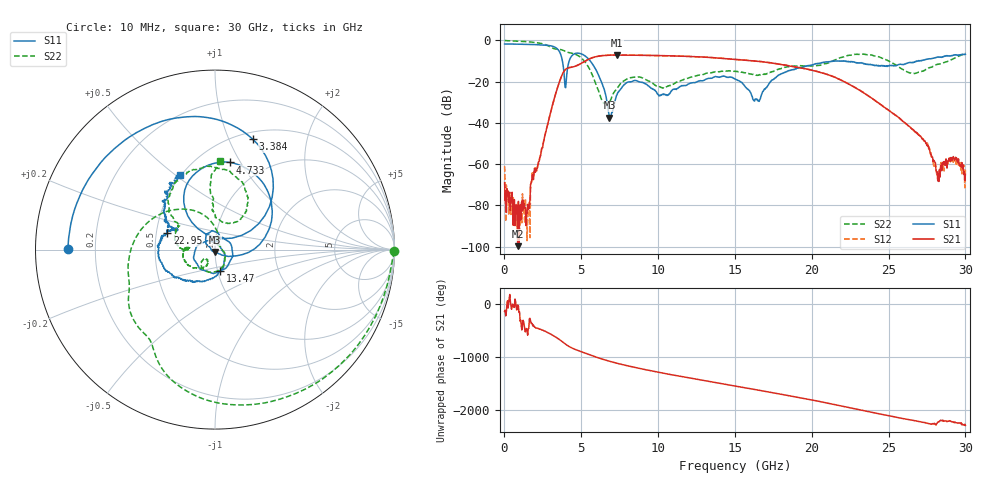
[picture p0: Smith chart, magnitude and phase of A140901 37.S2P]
!  2-Port S-parameters saved by WinCal
! VAR MeasName=S-Parameters (CALIBRATED_DATA) read from VNA (N5244A)
! VAR MeasDate=11/3/2014 9:33:30 AM
! VAR NAME=A140901 37
! VAR FILENAME=A140901 37.S2P
! VAR DATE=11/3/2014 9:33:30 AM
! VAR PHYS_PORTS=1,2
# Hz S RI R 50
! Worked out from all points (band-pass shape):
!   801 points, 10 MHz to 30 GHz, reference 50 ohm
!   highest |S21| = -7.08 dB at 7.32 GHz (marker M1); lowest = -99.8 dB at 872.2 MHz (marker M2)
!   |S21| within 3 dB of the highest: 5.239 GHz to 16.4 GHz (11.16 GHz wide, 103 % of centre)
!   lowest |S11| = -37.5 dB at 6.833 GHz (marker M3), VSWR 1.03, Z = 49.9 - j1.33 ohm
!   |S11| at or under -10 dB: 3.772 GHz to 4.21 GHz (438.1 MHz wide, 11 % of centre); 5.587 GHz to 21.47 GHz (15.89 GHz wide, 117 % of centre); 22.11 GHz to 26.84 GHz (4.729 GHz wide, 19.3 % of centre)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
!   |S22| runs from -30.6 to 0.0 dB; largest |S21 - S12| = 0.0029
!   S11 on the Smith chart (normalised r, x): 10 MHz: 0.10, +0.00; 3.384 GHz: 0.58, +1.23; 4.733 GHz: 0.70, +0.90; 13.47 GHz: 1.03, -0.25; 22.95 GHz: 0.57, +0.11; 30 GHz: 0.49, +0.52
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1e7  -0.8182 0.00205  -0.000212 -0.000286  -0.000372 0.000815  0.9981 -0.00942
8.722125e8  -0.7617 0.2785  1.02e-05 -1.47e-06  -4.44e-05 -8.61e-05  0.8121 -0.5097
1.5095e9  -0.6519 0.4648  -7.83e-05 6.98e-05  1.36e-06 4.44e-05  0.5214 -0.7674
3.383875e9  0.2098 0.6155  -0.00359 0.0589  -0.00398 0.0589  -0.3777 -0.4849
3.983675e9  -0.0108 0.0707  0.1672 -0.1095  0.1674 -0.109  -0.4805 -0.2445
4.733425e9  0.0835 0.4857  -0.2049 -0.139  -0.2044 -0.139  -0.4326 0.0811
5.033325e9  0.2457 0.3968  -0.2832 -0.00788  -0.2831 -0.00857  -0.3111 0.1942
5.933025e9  0.2011 -0.00685  0.0236 0.4008  0.0235 0.4011  0.014 0.0886
6.832725e9  -0.000875 -0.0133  0.4381 0.037  0.4381 0.0376  0.0307 0.0106
7.320062e9  -0.0412 0.0243  0.3702 -0.2429  0.3698 -0.242  0.0567 -0.038
1.001916e10  0.0183 0.0442  -0.3935 0.1743  -0.3929 0.1735  -0.0578 -0.0527
1.148118e10  0.0389 0.0665  0.099 0.4027  0.0981 0.4024  -0.051 -0.0932
1.346801e10  0.0299 -0.1172  0.3403 -0.1783  0.3404 -0.1775  -0.1365 -0.0918
1.5005e10  -0.1147 -0.0185  -0.0917 -0.3345  -0.0916 -0.3339  -0.1767 -0.0164
1.65045e10  0.0306 0.0188  -0.3106 0.0107  -0.3122 0.0101  -0.1446 0.01
2.002832e10  -0.199 -0.158  0.1856 -0.033  0.1869 -0.0327  -0.1974 0.1321
2.295235e10  -0.2658 0.0904  -0.0669 0.00637  -0.0668 0.00654  -0.1214 0.4461
2.501416e10  -0.2101 0.1136  0.0124 0.0158  0.0125 0.0159  0.1835 0.2603
2.73009e10  -0.2795 0.1858  0.000969 -0.00365  0.000977 -0.00362  0.000949 0.1866
2.82006e10  -0.2939 0.2705  0.000149 -0.000365  9.42e-05 -0.000439  -0.0171 0.2644
2.928774e10  -0.2449 0.373  0.000225 -0.0012  0.000419 -0.00125  -0.0246 0.3693
3e10  -0.1965 0.4169  -0.000382 -0.000419  -0.000558 -0.000476  0.0281 0.4932
